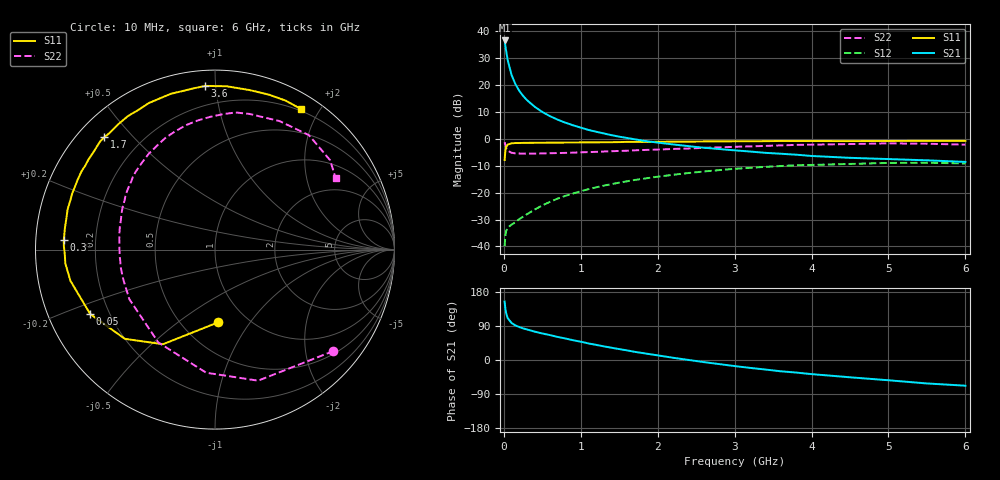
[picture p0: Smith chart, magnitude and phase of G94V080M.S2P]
! SIEMENS Small Signal Semiconductors
! BFG235
! Si NPN RF Bipolar Junction Transistor in SOT223
! VCE = 4 V  IC = 80 mA
! Common Emitter S-Parameters:  July  1994
# GHz  S  MA  R  50
!  f  S11  S21  S12  S22
! GHz  MAG  ANG  MAG  ANG  MAG  ANG  MAG  ANG
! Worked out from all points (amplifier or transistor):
!   40 points, 10 MHz to 6 GHz, reference 50 ohm
!   highest |S21| = 36.6 dB at 10 MHz (marker M1)
!   |S21| within 3 dB of that: start of sweep to 25.49 MHz
!   unconditionally stable (mu >= 1): 480.4 MHz to 1.441 GHz
!   at 200 MHz: K = 0.75, MSG = 23.9 dB, |S12| = -29.8 dB
!   at 1.5 GHz: K = 0.99, MSG = 8.6 dB, |S12| = -16.3 dB
!   at 6 GHz: K = 0.91, MSG = 0.3 dB, |S12| = -9.1 dB
!   S11 on the Smith chart (normalised r, x): 10 MHz: 0.74, -0.72; 50 MHz: 0.13, -0.24; 300 MHz: 0.08, +0.03; 1.7 GHz: 0.08, +0.42; 3.6 GHz: 0.08, +0.94; 6 GHz: 0.18, +1.78
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0.01  0.4053 -87.4  67.68 154.1  0.0101 65.1  0.8686 -40.6
0.02  0.6016 -118.8  54.24 135.7  0.016 50.4  0.7688 -71.8
0.03  0.7067 -135.3  43.27 123.6  0.0193 42.4  0.6877 -94.1
0.05  0.7824 -152.7  29.22 110.6  0.0225 33.5  0.6061 -121.4
0.1  0.824 -167.8  15.53 97.7  0.0254 33.3  0.5515 -149.9
0.15  0.8374 -174.7  10.46 91.2  0.0281 38.8  0.5374 -161.9
0.2  0.8373 -178.1  7.837 87.1  0.0322 43.1  0.5346 -168.6
0.25  0.8425 178.5  6.317 83.4  0.0357 46.5  0.5317 -173.1
0.3  0.8441 176.3  5.267 80.6  0.0396 49.6  0.5326 -176.9
0.4  0.8448 171.8  3.967 74.9  0.0484 53.0  0.5327 177.9
0.5  0.8464 167.8  3.167 70.0  0.0578 54.8  0.5365 173.6
0.6  0.8512 164.8  2.645 65.7  0.0675 55.5  0.5408 169.8
0.8  0.8548 158.5  2 56.7  0.0872 54.7  0.5488 163.1
1.1  0.8623 149.4  1.466 43.7  0.116 50.7  0.5682 154.3
1.4  0.8669 141.9  1.171 32.3  0.144 45.3  0.5891 146.1
1.7  0.8784 134.5  0.982 21.6  0.1721 39.4  0.6124 138.2
2.2  0.8881 123.2  0.788 5.9  0.2147 28.6  0.6493 124.6
3.2  0.9017 101.7  0.582 -20.8  0.2898 5.3  0.725 98.0
3.6  0.9137 93.4  0.529 -29.8  0.3124 -4.7  0.7561 86.6
4.5  0.9095 77.7  0.444 -45.6  0.3417 -24.8  0.8013 63.3
5.5  0.9187 64.6  0.399 -61.9  0.3596 -46.9  0.8119 37.8
6  0.9181 58.4  0.373 -67.8  0.3494 -55.0  0.781 30.5
